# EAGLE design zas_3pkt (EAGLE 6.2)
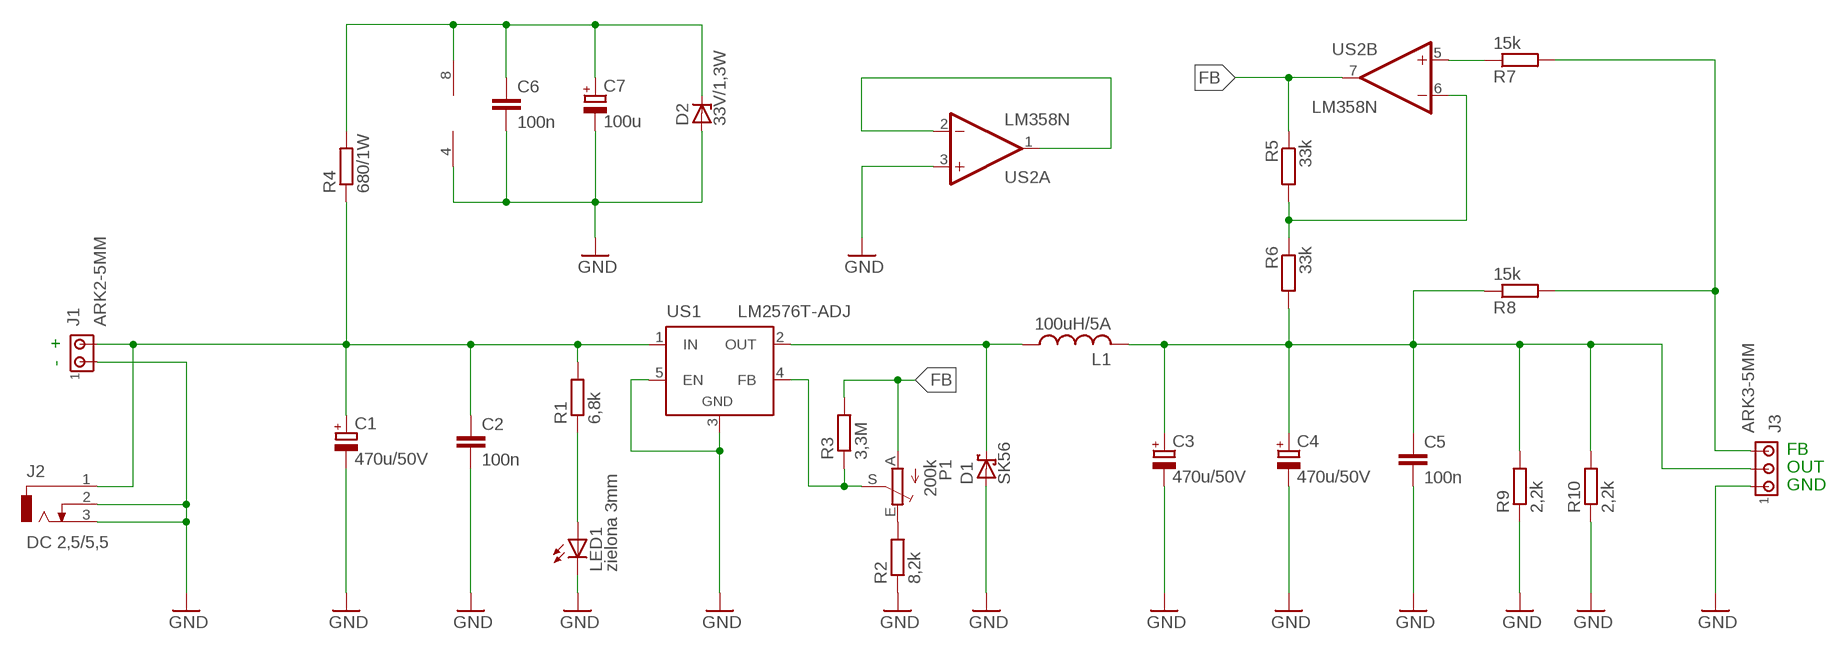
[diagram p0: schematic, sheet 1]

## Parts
C1  470u/50V  CPOL-EUE5-10.5  [E5-10,5]
C2  100n  C-EUC1206  [C1206]
C3  470u/50V  CPOL-EUE5-10.5  [E5-10,5]
C4  470u/50V  CPOL-EUE5-10.5  [E5-10,5]
C5  100n  C-EUC1206  [C1206]
C6  100n  C-EUC1206  [C1206]
C7  100u  CPOL-EUE2.5-6  [E2,5-6]
D1  SK56  SCHOTTKY-DIODESMD  [SMB]
D2  33V/1,3W  ZPY  [DO41Z10]
J1  ARK2-5MM  [2PIN-5MM]
J2  DC 2,5/5,5  DCJ0303  [DCJ0303]
J3  ARK3-5MM  [3PIN-5MM]
L1  100uH/5A  L-USTJ6-U1  [TJ6-U1]
LED1  zielona 3mm  LED3MM  [LED3MM]
P1  200k  TRIM_EU-CA6V  [CA6V]
R1  6,8k  R-EU_M1206  [M1206]
R2  8,2k  R-EU_M1206  [M1206]
R3  3,3M  R-EU_M1206  [M1206]
R4  680/1W  R-EU_0414/5V  [0414V]
R5  33k  R-EU_M1206  [M1206]
R6  33k  R-EU_M1206  [M1206]
R7  15k  R-EU_M1206  [M1206]
R8  15k  R-EU_M1206  [M1206]
R9  2,2k  R-EU_M1206  [M1206]
R10  2,2k  R-EU_M1206  [M1206]
US1  LM2576T-ADJ  LM2596TV  [TO220-51]
US2  LM358N  [DIL08]

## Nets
FB: P1.A R3.2 R5.1 US2.7(B:OUT)
GND: C1.- C2.2 C3.- C4.- C5.2 C6.2 C7.- D1.A D2.A J1.P$1 J2.2 J2.3 J3.P$1 LED1.K(C) R2.1 R9.1 R10.1 US1.3(GND) US1.5(EN) US2.3(A:+IN) US2.4(P:V-)
N$1: C1.+ C2.1 J1.P$2 J2.1 R1.2 R4.1 US1.1(IN)
N$2: D1.C L1.1 US1.2(OUT)
N$3: P1.E R2.2
N$4: LED1.A R1.1
N$5: C3.+ C4.+ C5.1 J3.P$2 L1.2 R6.2 R8.1 R9.2 R10.2
N$6: US2.1(A:OUT) US2.2(A:-IN)
N$7: R5.2 R6.1 US2.6(B:-IN)
N$9: J3.P$3 R7.2 R8.2
N$10: P1.S R3.1 US1.4(FB)
N$11: C6.1 C7.+ D2.C R4.2 US2.8(P:V+)
N$12: R7.1 US2.5(B:+IN)

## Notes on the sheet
- +
- -
- FB
- OUT
- GND

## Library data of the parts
C1 C3 C4 C7 = rcl:CPOL-EU: POLARIZED CAPACITOR, European symbol
C2 C5 C6 = rcl:C-EU: CAPACITOR, European symbol
D1 = diode:SCHOTTKY-DIODE: Schottky Diode
D2 = diode:ZPY: Z DIODE
J1 = zlacza_futrzak:ARK2: ARK 2
J2 = con-jack:DCJ0303: DC POWER JACK Source: DCJ0303.pdf; OC_FARNELL: unknown; OC_NEWARK: unknown
J3 = zlacza_futrzak:ARK3: ARK 3 Raster 5mm i 3,5mm
L1 = rcl:L-US: INDUCTOR, American symbol
LED1 = led:LED: LED
P1 = pot:TRIM_EU-: POTENTIOMETER
R1-R10 = rcl:R-EU_: RESISTOR, European symbol
US1 = linear:LM2596T: STEP-DOWN VOLTAGE REGULATOR
US2 = linear:LM358: OP AMP also LM158; LM258; LM2904 Source: http://cache.national.com/ds/LM/LM158.pdf

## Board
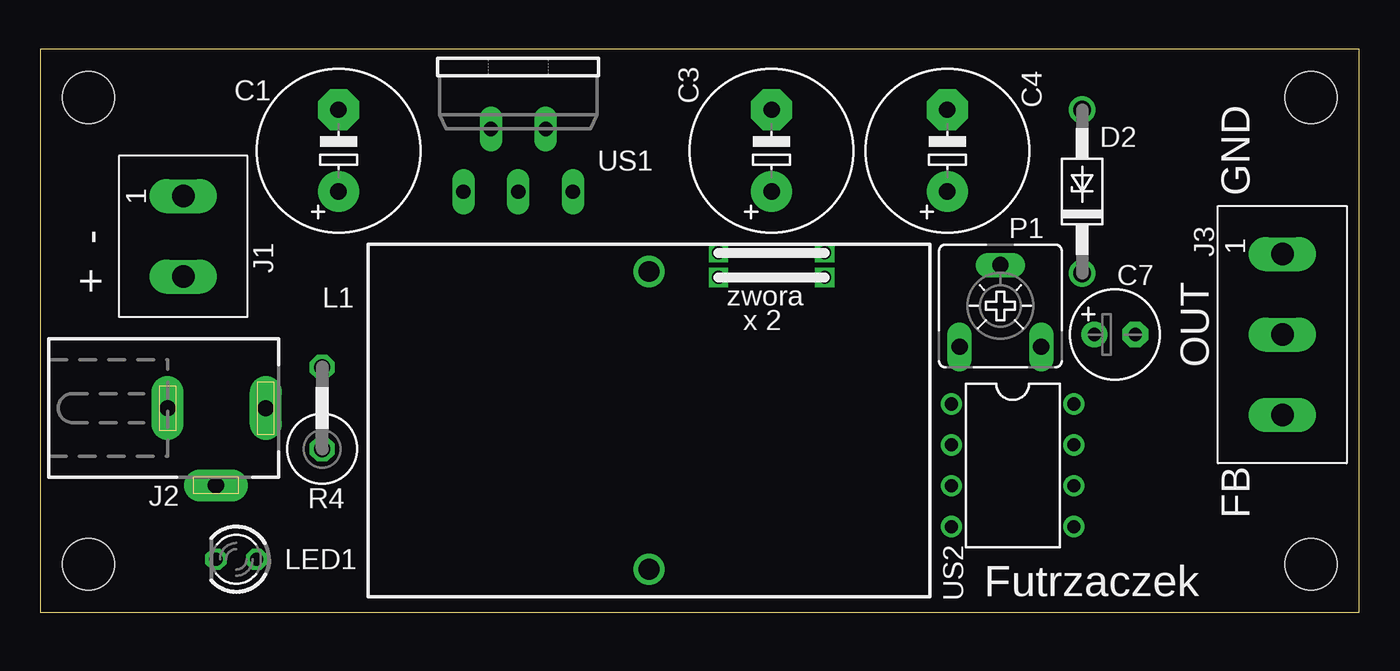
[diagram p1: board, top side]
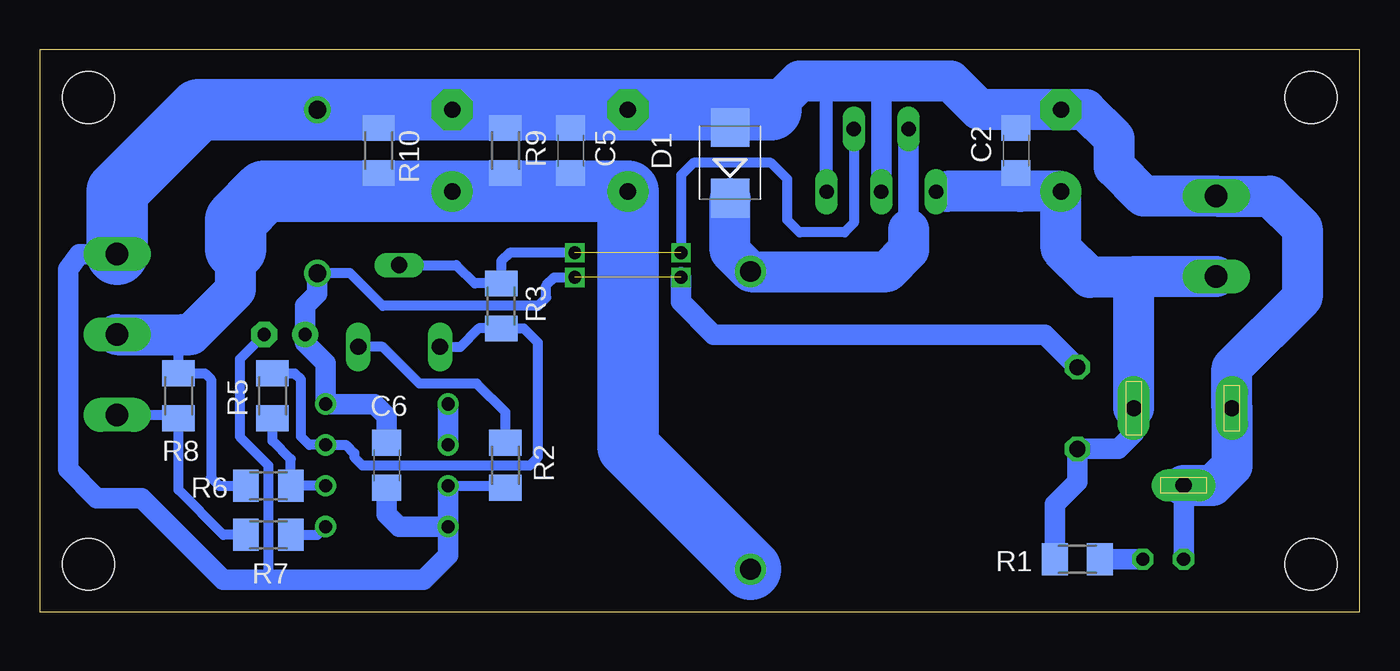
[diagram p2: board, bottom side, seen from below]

Size 82 x 35 mm. Coordinates in mm from the lower left corner, seen from the top.
Outline: 0,0 82,0 82,35 0,35 0,0
Copper layers (1*16): Top 0.035mm / dielectric 1.5mm / Bottom 0.035mm
Design rules: minimum track width 10mil, minimum drill 24mil, track to track 8mil, track to pad 8mil, pad to pad 8mil, via to via 8mil, smd to smd 8mil, copper to edge 40mil, drill to drill 8mil, minimum pad ring 10mil, minimum via ring 8mil, stop-mask expansion 4mil, vias tented up to drill 0mil, thermal gap 10mil
Holes 3.2 mm at 3,32 3,3 79,3 79,32

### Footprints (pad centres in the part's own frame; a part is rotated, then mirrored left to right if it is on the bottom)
E5-10,5 = drill 1.016 pad 2.54: + -2.54,0 | drill 1.016 pad 2.54 octagon: - 2.54,0
C1206 = smd 1.6 x 1.8: 1 -1.4,0; 2 1.4,0
E2,5-6 = drill 0.813 pad 1.6: + -1.27,0 | drill 0.813 pad 1.6 octagon: - 1.27,0
SMB = smd 2.4 x 2.4: A 2.2,0; C -2.2,0
DO41Z10 = drill 1.118: A 5.08,0; C -5.08,0
2PIN-5MM = drill 1.4 long: P$1 -2.5,0; P$2 2.5,0
DCJ0303 = drill 1 pad 2 long: 1 0,3.1; 2 4.8,0; 3 0,-3
3PIN-5MM = drill 1.4 long: P$1 -5,0; P$2 0,0; P$3 5,0
TJ6-U1 = drill 1.3: 1 -9.25,0; 2 9.25,0
LED3MM = drill 0.813 octagon: A -1.27,0; K 1.27,0
CA6V = drill 1.016 long: A -2.54,-2.54; E 2.54,-2.54; S 0,2.54
M1206 = smd 1.6 x 2: 1 -1.4,0; 2 1.4,0
0414V = drill 1.016 octagon: 1 -2.54,0; 2 2.54,0
TO220-51 = drill 0.9 long: 1 -3.4,-8.4; 2 -1.7,-4.5; 3 0,-8.4; 4 1.7,-4.5; 5 3.4,-8.4
DIL08 = drill 0.813 pad 1.27: 1 -3.81,-3.81; 2 -1.27,-3.81; 3 1.27,-3.81; 4 3.81,-3.81; 5 3.81,3.81; 6 1.27,3.81; 7 -1.27,3.81; 8 -3.81,3.81

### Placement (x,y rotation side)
C1  18.54,28.7 90 top
C2  21.34,28.7 90 bottom
C3  45.47,28.7 90 top
C4  56.39,28.7 90 top
C5  49.02,28.7 90 bottom
C6  60.45,9.14 270 bottom
C7  66.8,17.27 0 top
D1  39.12,27.94 90 bottom
D2  64.77,26.16 90 top
J1  8.89,23.37 270 top
J2  10.92,12.7 270 top
J3  77.22,17.27 270 top
L1  37.85,11.94 270 top
LED1  12.19,3.3 180 top
P1  59.69,19.05 0 top
R1  17.53,3.3 180 bottom
R2  53.09,9.14 90 bottom
R3  53.34,19.05 270 bottom
R4  17.53,12.7 90 top
R5  67.56,13.46 270 bottom
R6  67.82,7.87 180 bottom
R7  67.82,4.83 180 bottom
R8  73.41,13.46 270 bottom
R9  53.09,28.7 270 bottom
R10  60.96,28.7 270 bottom
US1  29.72,34.54 0 top
US2  60.45,9.14 270 top

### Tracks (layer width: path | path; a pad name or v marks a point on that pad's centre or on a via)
FB
  Bottom 0.61: P1.A 55.88,16.51 54.74,17.65 R3.2 51.94,17.65 51.05,16.76 51.05,9.65 51.56,9.14 61.98,9.14 62.48,9.65 62.48,9.91 62.99,10.41 US2.7 65.28,10.41 65.79,10.92 65.79,14.48 66.17,14.86 R5.1
GND
  Bottom 0.61: US2.3 53.22,7.87 R2.1 | C7.- 69.6,15.75 69.6,10.92 67.82,9.14 67.82,2.03
  Bottom 0.813: US1.5 33.12,32.92 33.02,33.02
  Bottom 1.27: US1.3 29.72,32.77 29.97,33.02 | C2.2 21.34,31.24 | D1.A 39.01,31.39 38.86,31.24 | 33.12,32.67 32.77,33.02 | LED1.K J2.2 | C6.2 60.45,6.1 59.69,5.33 US2.4 | US2.4 56.64,3.56 58.17,2.03 67.82,2.03 70.61,2.03 75.69,7.11 78.49,7.11 80.26,8.89 80.26,21.34 79.58,22.27 J3.P$1 | US2.3 US2.4 | C5.2 49.02,31.24 | R9.1 53.09,31.24 53.09,31.75 | R10.1 60.96,30.99 61.21,31.24
  Bottom 2.54: 36.58,31.24 34.8,33.02 33.02,33.02 32.77,33.02 29.97,33.02 25.4,33.02 23.62,31.24 21.34,31.24 C1.- 17.02,31.24 15.24,29.46 15.24,27.69 13.42,25.87 J1.P$1 5.55,25.87 3.56,23.88 3.56,19.56 7.92,15.19 J2.3 7.92,9.1 9.12,7.9 J2.2
  Bottom 3.81: 36.58,31.24 38.86,31.24 C3.- 49.02,31.24 53.09,31.24 C4.- 61.21,31.24 D2.A 72.14,31.24 77.22,26.16 J3.P$1
N$1
  Bottom 1.27: 25.65,26.16 26.05,26.16 US1.1 | C2.1 21.34,26.42 21.08,26.16 | J2.1 14.02,11.12 14.99,10.16 R4.1 17.53,8.13 18.93,6.73 R1.2
  Bottom 2.54: 25.65,26.16 21.08,26.16 C1.+ 18.54,22.61 16.76,20.83 14.02,20.83 | J2.1 14.02,20.83 | J1.P$2 13.98,20.87 14.02,20.83
N$2
  Bottom 1.27: US1.2 28.02,23.8
  Bottom 2.54: 28.02,23.8 28.02,22.53 29.36,21.19 L1.1 39.12,22.46 D1.C
N$3
  Bottom 0.61: R2.2 53.09,12.45 54.86,14.22 58.42,14.22 60.71,16.51 P1.E
N$4
  Bottom 1.27: R1.1 LED1.A
N$5
  Bottom 0.61: 73.15,17.27 73.41,17.02 R8.1 71.76,14.86 71.37,14.48 71.37,8.38 70.87,7.87 R6.2
  Bottom 1.27: C5.1 49.02,26.16 | R9.2 53.09,26.16 | R10.2 60.96,26.16
  Bottom 2.54: 69.85,22.61 69.85,20.07 72.64,17.27 73.15,17.27 J3.P$2
  Bottom 3.81: L1.2 45.47,10.31 C3.+ 49.02,26.16 53.09,26.16 C4.+ 60.96,26.16 68.07,26.16 69.85,24.38 69.85,22.61
N$6
  Bottom 1.27: US2.1 US2.2
N$7
  Bottom 0.61: R5.2 67.56,10.67 66.42,9.52 R6.1 US2.6
N$9
  Bottom 0.61: J3.P$3 73.62,12.27 R8.2 73.41,7.62 70.61,4.83 R7.2
N$10  (via drill 0.8)  (1 unrouted)
  Bottom 0.61: US1.4 31.42,24.21 32,23.62 34.8,23.62 35.56,24.38 35.56,26.92 36.58,27.94 41.4,27.94 42.16,27.18 v42.16,22.35 | P1.S 56.13,21.59 54.99,20.45 R3.1 53.34,21.84 52.83,22.35 v48.77,22.35
N$11  (via drill 0.8)  (1 unrouted)
  Bottom 0.61: v48.77,20.83 50.04,20.83 50.55,20.32 50.55,19.56 51.05,19.05 60.71,19.05 62.74,21.08 D2.C
  Bottom 1.27: R4.2 19.56,17.27 40.13,17.27 42.16,19.3 v42.16,20.83 | C6.1 60.45,12.19 61.21,12.95 US2.8 64.26,15.49 65.53,16.76 C7.+ 65.53,19.05 64.77,19.81 D2.C
N$12
  Bottom 0.61: R7.1 64.77,4.83 US2.5

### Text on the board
tPlace: GND | + - | zwora | x 2 | OUT | FB | Futrzaczek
